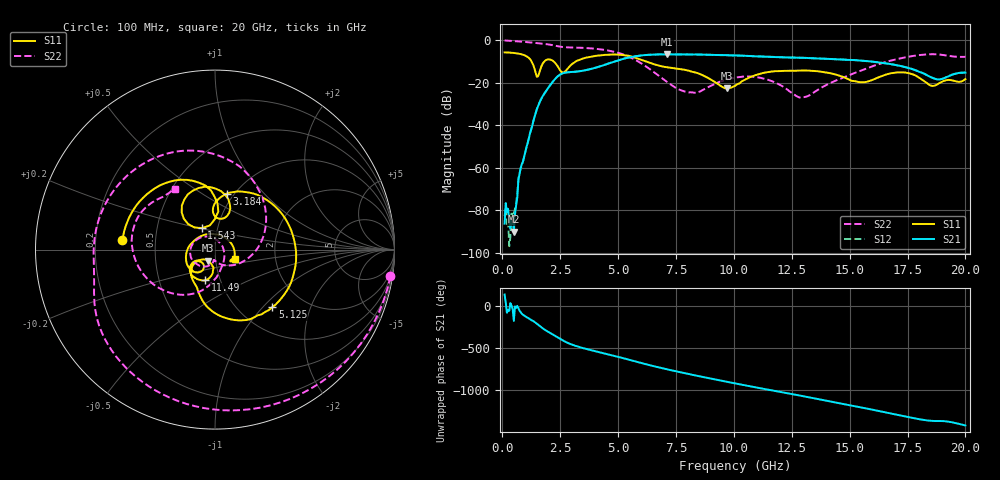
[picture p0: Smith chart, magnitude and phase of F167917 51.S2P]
!  2-Port S-parameters saved by WinCal
! VAR MeasName=S-Parameters (CALIBRATED_DATA) read from VNA (N5242A)
! VAR MeasDate=2016-11-22 9:02:24
! VAR NAME=F167917 51
! VAR FILENAME=F167917 51.S2P
! VAR DATE=2016-11-22 9:02:24
! VAR PHYS_PORTS=1,2
# Hz S DB R 50
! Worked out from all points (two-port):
!   401 points, 100 MHz to 20 GHz, reference 50 ohm
!   highest |S21| = -6.64 dB at 7.115 GHz (marker M1); lowest = -90.2 dB at 498 MHz (marker M2)
!   |S21| within 3 dB of the highest: 4.974 GHz to 15.53 GHz (10.55 GHz wide, 103 % of centre)
!   lowest |S11| = -22.6 dB at 9.702 GHz (marker M3), VSWR 1.16, Z = 45.9 - j5.75 ohm
!   |S11| at or under -10 dB: 1.263 GHz to 1.814 GHz (551.4 MHz wide, 35.8 % of centre); 2.221 GHz to 3.173 GHz (952.1 MHz wide, 35.3 % of centre); 6.206 GHz to end of sweep
!   |S22| runs from -27.0 to -0.1 dB; largest |S21 - S12| = 0.004
!   S11 on the Smith chart (normalised r, x): 100 MHz: 0.32, +0.05; 1.543 GHz: 0.84, +0.21; 3.184 GHz: 0.93, +0.64; 5.125 GHz: 1.40, -1.13; 11.49 GHz: 0.85, -0.30; 20 GHz: 1.24, -0.13
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1e8  -5.71 174.2  -86.33 141.8  -82.78 48.7  -0.10 -8.7
4.98e8  -5.98 150.5  -90.20 -171.9  -81.26 -45.3  -0.37 -40.7
7.965e8  -6.51 131.2  -60.03 -68.8  -60.24 -74.3  -0.62 -63.2
1.54275e9  -17.03 121.6  -31.02 142.2  -31.01 142.5  -1.39 -112.7
1.94075e9  -9.09 110.4  -23.11 64.3  -23.10 64.3  -1.89 -135.6
2.3885e9  -12.22 69.6  -17.04 -8.8  -17.05 -8.8  -2.79 -158.2
3.1845e9  -9.92 78.1  -14.80 -111.5  -14.79 -111.6  -3.45 171.1
3.43325e9  -8.79 61.9  -14.43 -132.2  -14.43 -132.2  -3.55 160.4
4.32875e9  -7.01 4.5  -11.94 165.9  -11.93 165.9  -4.41 118.4
5.12475e9  -6.87 -45.2  -9.12 111.1  -9.13 111.3  -6.29 73.9
5.871e9  -8.68 -86.2  -7.37 55.7  -7.33 55.8  -10.01 26.2
6.7665e9  -11.96 -111.6  -6.67 -6.7  -6.65 -6.7  -16.78 -34.8
7.11475e9  -12.72 -116.5  -6.64 -29.1  -6.62 -29.1  -19.65 -57.0
8.30875e9  -15.14 -138.2  -6.69 -100.0  -6.65 -100.0  -24.71 -97.5
9.70175e9  -22.64 -122.3  -7.04 -177.6  -7.03 -177.5  -18.40 -129.2
1.005e10  -21.47 -103.0  -7.14 163.6  -7.15 163.7  -17.67 -143.0
1.149275e10  -14.96 -107.4  -7.81 88.1  -7.75 88.0  -18.70 151.8
1.338325e10  -14.41 -134.6  -8.46 -9.6  -8.42 -9.7  -25.11 -21.5
1.497525e10  -18.51 -149.0  -9.28 -93.4  -9.24 -93.7  -16.41 -86.1
1.67165e10  -15.73 -129.1  -11.11 168.6  -11.15 168.6  -9.76 -129.8
1.835825e10  -20.39 116.0  -16.56 81.2  -16.51 81.3  -6.61 174.0
2e10  -18.31 -24.3  -15.25 22.1  -15.16 22.4  -7.82 123.7
